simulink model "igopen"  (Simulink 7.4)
settings: Solver=ode45  StartTime=0  StopTime=20  MaxStep=1e-3  RelTol=1e-3
undefined symbols (not defined in the file or in its folder): sat

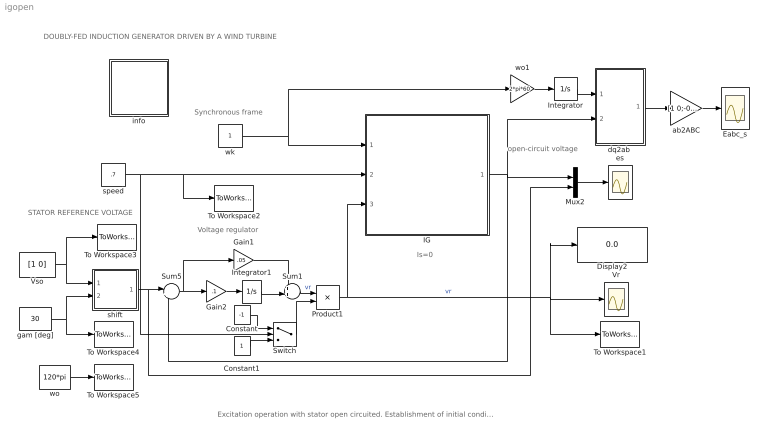
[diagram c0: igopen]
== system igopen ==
  note: STATOR REFERENCE VOLTAGE
  note: Synchronous frame
  note: DOUBLY-FED INDUCTION GENERATOR DRIVEN BY A WIND TURBINE
  note: Excitation operation with stator open circuited. Establishment of initial conditions.
  note: Is=0
  note: open-circuit voltage
  note: Voltage regulator
  Constant : Constant  Value=-1  OutDataType=sfix(16)  OutScaling=2^0
  Constant1 : Constant  OutDataType=sfix(16)  OutScaling=2^0
  Display2 : Display
  Eabc_s : Scope
  Gain1 : Gain  Gain=.05  ParameterDataType=sfix(16)  ParameterScaling=2^0  OutDataType=sfix(16)  OutScaling=2^0
  Gain2 : Gain  Gain=.1  ParameterDataType=sfix(16)  ParameterScaling=2^0  OutDataType=sfix(16)  OutScaling=2^0
  IG : Subsystem  mask{Rr=.02, Lm=5, Lrl=0.1, wo=2*pi*60}
      mask prompts: Rr "Rotor resistance [pu]"; Lm "Magnetizing inductance [pu]"; Lrl "Rotor leakage inductance [pu]"; wo "base frequency [rad/s]"
  Integrator : Integrator
  Integrator1 : Integrator  UpperSaturationLimit=sat  LowerSaturationLimit=-sat
  Mux2 : Mux  Inputs=2
  Product1 : Product  OutDataType=sfix(16)  OutScaling=2^0
  Sum1 : Sum  Inputs=++|  OutDataType=sfix(16)  OutScaling=2^0
  Sum5 : Sum  Inputs=|+-  OutDataType=sfix(16)  OutScaling=2^0
  Switch : Switch  Criteria=u2 > Threshold  Threshold=1
  To Workspace1 : ToWorkspace  VariableName=vro  SampleTime=-1  SaveFormat=Array
  To Workspace2 : ToWorkspace  VariableName=wmo  SampleTime=-1  SaveFormat=Array
  To Workspace3 : ToWorkspace  VariableName=vso  SampleTime=-1  SaveFormat=Array
  To Workspace4 : ToWorkspace  VariableName=gamo  SampleTime=-1  SaveFormat=Array
  To Workspace5 : ToWorkspace  VariableName=wo  SampleTime=-1  SaveFormat=Array
  Vr : Scope
  Vso : Constant  Value=[1 0]  OutDataType=sfix(16)  OutScaling=2^0
  ab2ABC : Gain  Gain=[1 0;-0.5 sqrt(3)/2;-0.5 -sqrt(3)/2]  Multiplication=Matrix(K*u)  ParameterDataType=sfix(16)  ParameterScaling=2^0  OutDataType=sfix(16)  OutScaling=2^0
  "dq2ab " : Subsystem
  es : Scope
  gam [deg] : Constant  Value=30  OutDataType=sfix(16)  OutScaling=2^0
  info : Subsystem
  shift : Subsystem
  speed : Constant  Value=.7  OutDataType=sfix(16)  OutScaling=2^0
  wk : Constant  OutDataType=sfix(16)  OutScaling=2^0
  wo : Constant  Value=120*pi  OutDataType=sfix(16)  OutScaling=2^0
  wo1 : Gain  Gain=2*pi*60  ParameterDataType=sfix(16)  ParameterScaling=2^0  OutDataType=sfix(16)  OutScaling=2^0
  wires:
  IG/1(es) -> Sum5/2, Mux2/1, "dq2ab "/2(dq)
  Sum5/1 -> Gain2/1, Gain1/1
  speed/1 -> IG/2(wm), To Workspace2/1, Switch/2
  wk/1 -> IG/1(wk), wo1/1
  Vso/1 -> shift/1(vso), To Workspace3/1
  gam [deg]/1 -> shift/2(gama), To Workspace4/1
  wo/1 -> To Workspace5/1
  Gain2/1 -> Integrator1/1
  shift/1(vs) -> Sum5/1, Mux2/2
  Mux2/1 -> es/1
  Integrator1/1 -> Sum1/2
  Gain1/1 -> Sum1/1
  Constant/1 -> Switch/1
  Constant1/1 -> Switch/3
  Sum1/1 -> Product1/1  "vr"
  Product1/1 -> IG/3(vr), Vr/1, Display2/1, To Workspace1/1  "vr"
  Switch/1 -> Product1/2
  "dq2ab "/1(ab) -> ab2ABC/1
  ab2ABC/1 -> Eabc_s/1
  wo1/1 -> Integrator/1
  Integrator/1 -> "dq2ab "/1(thetas)

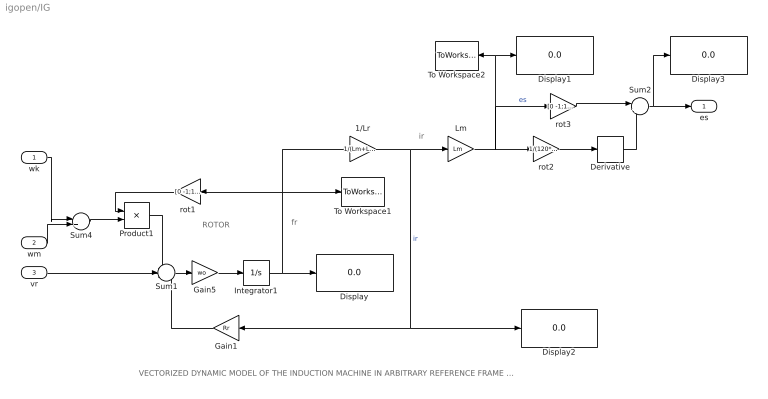
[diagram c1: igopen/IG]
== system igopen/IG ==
  note: ROTOR
  note: fr
  note: VECTORIZED DYNAMIC MODEL OF THE INDUCTION MACHINE IN ARBITRARY REFERENCE FRAME (stator open circuited --is=0)
  note: ir
  wk : Inport  OutDataType=sfix(16)  OutScaling=2^0
  wm : Inport  Port=2  OutDataType=sfix(16)  OutScaling=2^0
  vr : Inport  Port=3  OutDataType=sfix(16)  OutScaling=2^0
  1/Lr : Gain  Gain=1/(Lm+Lrl)  ParameterDataType=sfix(16)  ParameterScaling=2^0  OutDataType=sfix(16)  OutScaling=2^0
  Derivative : Derivative
  Display{,1..3} (4 alike) : Display
  Gain1 : Gain  Gain=Rr  ParameterDataType=sfix(16)  ParameterScaling=2^0  OutDataType=sfix(16)  OutScaling=2^0
  Gain5 : Gain  Gain=wo  ParameterDataType=sfix(16)  ParameterScaling=2^0  OutDataType=sfix(16)  OutScaling=2^0
  Integrator1 : Integrator  InitialCondition=[0 -1]
  Lm : Gain  Gain=Lm  ParameterDataType=sfix(16)  ParameterScaling=2^0  OutDataType=sfix(16)  OutScaling=2^0
  Product1 : Product  OutDataType=sfix(16)  OutScaling=2^0
  Sum1 : Sum  Inputs=-+-  OutDataType=sfix(16)  OutScaling=2^0
  Sum2 : Sum  Inputs=|++  OutDataType=sfix(16)  OutScaling=2^0
  Sum4 : Sum  Inputs=|+-  OutDataType=sfix(16)  OutScaling=2^0
  To Workspace1 : ToWorkspace  VariableName=fro  SampleTime=-1  SaveFormat=Array
  To Workspace2 : ToWorkspace  VariableName=fso  SampleTime=-1  SaveFormat=Array
  rot1 : Gain  Gain=[0 -1;1 0]  Multiplication=Matrix(K*u)  ParameterDataType=sfix(16)  ParameterScaling=2^0  OutDataType=sfix(16)  OutScaling=2^0
  rot2 : Gain  Gain=1/(120*pi)  Multiplication=Matrix(K*u)  ParameterDataType=sfix(16)  ParameterScaling=2^0  OutDataType=sfix(16)  OutScaling=2^0
  rot3 : Gain  Gain=[0 -1;1 0]  Multiplication=Matrix(K*u)  ParameterDataType=sfix(16)  ParameterScaling=2^0  OutDataType=sfix(16)  OutScaling=2^0
  es : Outport
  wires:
  Gain1/1 -> Sum1/3
  Integrator1/1 -> rot1/1, To Workspace1/1, 1/Lr/1, Display/1
  Product1/1 -> Sum1/1
  rot1/1 -> Product1/1
  Sum4/1 -> Product1/2
  Sum1/1 -> Gain5/1
  Gain5/1 -> Integrator1/1
  wk/1 -> Sum4/1
  wm/1 -> Sum4/2
  vr/1 -> Sum1/2
  Lm/1 -> Display1/1, To Workspace2/1, rot3/1, rot2/1  "es"
  Sum2/1 -> es/1, Display3/1
  rot3/1 -> Sum2/1
  Derivative/1 -> Sum2/2
  rot2/1 -> Derivative/1
  1/Lr/1 -> Lm/1, Gain1/1, Display2/1  "ir"

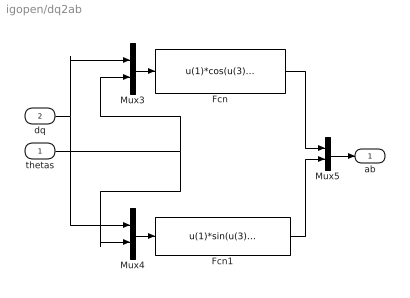
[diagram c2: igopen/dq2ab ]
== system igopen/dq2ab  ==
  thetas : Inport  OutDataType=sfix(16)  OutScaling=2^0
  dq : Inport  Port=2  OutDataType=sfix(16)  OutScaling=2^0
  Fcn : Fcn  Expr=u(1)*cos(u(3))-u(2)*sin(u(3))
  Fcn1 : Fcn  Expr=u(1)*sin(u(3))+u(2)*cos(u(3))
  Mux3 : Mux  Inputs=2
  Mux4 : Mux  Inputs=2
  Mux5 : Mux  Inputs=2
  ab : Outport
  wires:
  Mux3/1 -> Fcn/1
  Mux4/1 -> Fcn1/1
  dq/1 -> Mux3/1, Mux4/1
  thetas/1 -> Mux3/2, Mux4/2
  Fcn1/1 -> Mux5/2
  Fcn/1 -> Mux5/1
  Mux5/1 -> ab/1

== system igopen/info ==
  note: The induction machine runs at a specified speed with the stator disconnected from the grid (is=0). The rotor is suddenly excited with slip-frequency voltages derived from voltage regulators so as to produce a commanded open-circuit stator terminal voltage. The induction machine is modeled in vectorized form in the synchronous frame . The specified operating conditions and the final values of the variables reached in a dc steady state are all saved in the workspace to serve as initial conditions in a subsequent simulation. This simulation deals with the connection of the stator to the grid.
  note: Doubly-Fed Induction Generator driven by a Wind Turbine Stator disconnected from grid

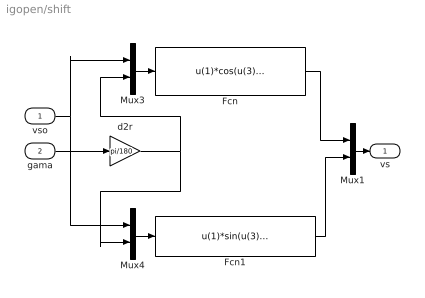
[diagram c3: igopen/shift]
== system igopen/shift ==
  vso : Inport  OutDataType=sfix(16)  OutScaling=2^0
  gama : Inport  Port=2  OutDataType=sfix(16)  OutScaling=2^0
  Fcn : Fcn  Expr=u(1)*cos(u(3))-u(2)*sin(u(3))
  Fcn1 : Fcn  Expr=u(1)*sin(u(3))+u(2)*cos(u(3))
  Mux1 : Mux  Inputs=2
  Mux3 : Mux  Inputs=2
  Mux4 : Mux  Inputs=2
  d2r : Gain  Gain=pi/180  Multiplication=Matrix(K*u)  ParameterDataType=sfix(16)  ParameterScaling=2^0  OutDataType=sfix(16)  OutScaling=2^0
  vs : Outport
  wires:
  Mux3/1 -> Fcn/1
  Mux4/1 -> Fcn1/1
  vso/1 -> Mux3/1, Mux4/1
  gama/1 -> d2r/1
  Fcn/1 -> Mux1/1
  Fcn1/1 -> Mux1/2
  d2r/1 -> Mux3/2, Mux4/2
  Mux1/1 -> vs/1
